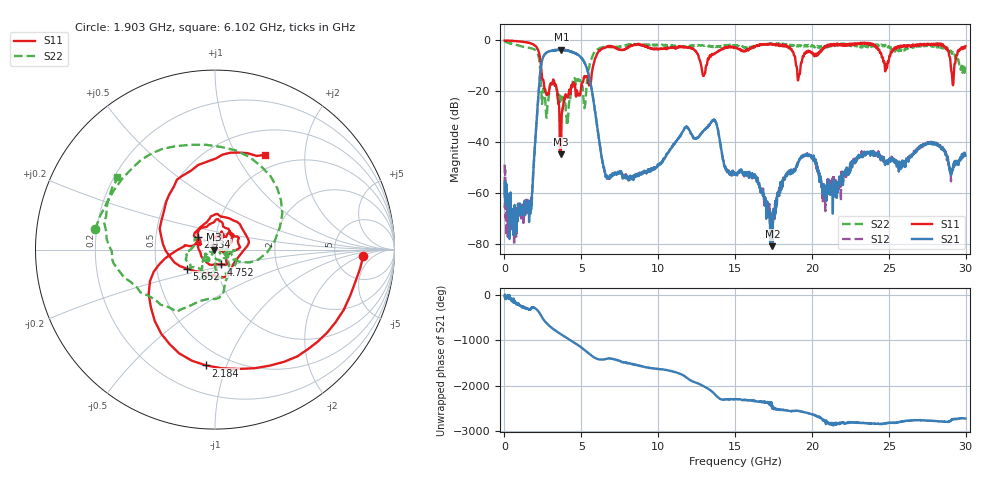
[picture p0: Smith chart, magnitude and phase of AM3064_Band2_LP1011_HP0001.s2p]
# Hz S DB R 50.0
!freq dBS11 angS11 dBS21 angS21 dBS12 angS12 dBS22 angS22
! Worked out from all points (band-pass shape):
!   1600 points, 10 MHz to 29.98 GHz, reference 50 ohm
!   highest |S21| = -3.61 dB at 3.703 GHz (marker M1); lowest = -80.9 dB at 17.42 GHz (marker M2)
!   |S21| within 3 dB of the highest: 2.517 GHz to 4.953 GHz (2.436 GHz wide, 65.2 % of centre)
!   lowest |S11| = -44.8 dB at 3.646 GHz (marker M3), VSWR 1.01, Z = 49.4 - j0.128 ohm
!   |S11| at or under -10 dB: 2.373 GHz to 5.771 GHz (3.397 GHz wide, 83.4 % of centre); 12.8 GHz to 13.12 GHz (319.9 MHz wide, 2.47 % of centre); 18.98 GHz to 19.27 GHz (289.7 MHz wide, 1.51 % of centre)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
!   |S22| runs from -33.4 to -0.3 dB; largest |S21 - S12| = 0.019
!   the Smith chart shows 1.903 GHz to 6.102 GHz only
!   S11 on the Smith chart (normalised r, x): 1.903 GHz: 10, -2; 2.184 GHz: 0.38, -0.85; 2.934 GHz: 0.82, +0.12; 4.752 GHz: 1.05, -0.17; 5.652 GHz: 0.72, -0.16; 6.102 GHz: 0.81, +1.33
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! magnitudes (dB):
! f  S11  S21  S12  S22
! 10 MHz  0.0  -55.6  -48.8  -0.3
! 609.8 MHz  -0.2  -70.1  -67.8  -1.5
! 1.641 GHz  -1.0  -64.2  -65.3  -3.0
! 1.903 GHz  -1.6  -48.9  -48.8  -3.4
! 2.184 GHz  -3.8  -23.5  -23.4  -5.5
! 2.597 GHz  -18.5  -5.7  -5.7  -22.1
! 2.934 GHz  -18.6  -4.3  -4.2  -18.9
! 3.646 GHz  -44.8  -3.6  -3.7  -24.9
! 3.703 GHz  -35.0  -3.6  -3.7  -22.0
! 4.752 GHz  -21.1  -5.6  -5.6  -15.9
! 5.015 GHz  -17.1  -7.1  -6.9  -18.3
! 5.652 GHz  -14.5  -18.4  -18.5  -7.3
! 6.102 GHz  -4.5  -37.0  -36.8  -3.4
! 6.739 GHz  -2.5  -53.9  -54.7  -2.3
! 10 GHz  -3.4  -49.2  -49.0  -1.9
! 13.6 GHz  -5.3  -31.5  -31.3  -2.6
! 15 GHz  -2.6  -52.9  -52.4  -1.8
! 17.42 GHz  -1.7  -80.9  -71.6  -1.4
! 19.99 GHz  -4.6  -45.8  -45.7  -1.9
! 20.83 GHz  -3.0  -59.5  -59.2  -2.4
! 25 GHz  -7.9  -47.5  -47.0  -2.3
! 29.98 GHz  -2.3  -45.4  -45.6  -10.4
